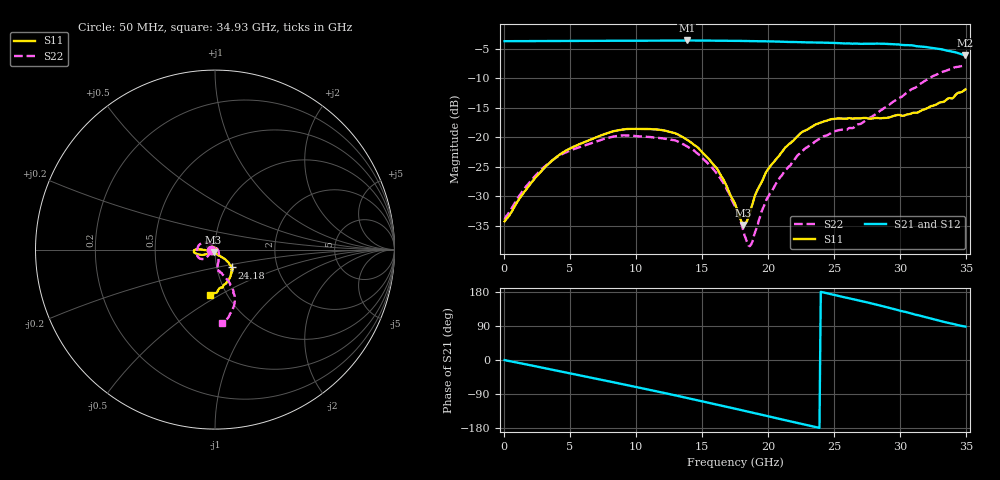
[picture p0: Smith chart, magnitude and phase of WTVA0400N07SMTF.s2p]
! 50 ohm 2-Port S-parameters measured by Modelithics Inc support@modelithics.com  Tampa, FL USA 813-866-6335 (February 2024)
! Smiths Interconnect,  4dB P/N: WTVA0400N07SMTF, Temperature: 50 C
! Board: 10 mil Rogers 4350B, Mounting Pad Dimensions: Length: 15 mils, Width: 25 mils, Gap: 40 mils.
# Hz S RI R 50
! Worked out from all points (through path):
!   352 points, 50 MHz to 34.93 GHz, reference 50 ohm
!   highest |S21| = -3.56 dB at 13.83 GHz (marker M1); lowest = -6.1 dB at 34.93 GHz (marker M2)
!   group delay of S21, straight-line fit = 21.7 ps
!   lowest |S11| = -34.9 dB at 18.11 GHz (marker M3), VSWR 1.04, Z = 49.2 - j1.58 ohm
!   |S11| at or under -10 dB: start of sweep to end of sweep
!   |S22| runs from -38.4 to -7.7 dB; largest |S21 - S12| = 0.0068
!   S11 on the Smith chart (normalised r, x): 50 MHz: 0.96, -0.00; 24.18 GHz: 1.18, -0.24; 34.93 GHz: 0.83, -0.45
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5e7  -0.0195 -0.000462  0.6541 -0.00359  0.6535 -0.00359  -0.0199 -0.00199
1.4935e9  -0.0301 -0.0157  0.6452 -0.1169  0.6447 -0.1168  -0.0289 -0.0217
2.8865e9  -0.0465 -0.0242  0.6176 -0.2259  0.6171 -0.2256  -0.0401 -0.0364
4.2795e9  -0.0662 -0.0293  0.5703 -0.3292  0.5696 -0.3291  -0.0531 -0.0472
5.8715e9  -0.0845 -0.0284  0.4946 -0.4358  0.4942 -0.4355  -0.0652 -0.0524
8.6575e9  -0.1135 -0.0182  0.3151 -0.5795  0.3141 -0.5792  -0.0944 -0.0416
1.1742e10  -0.1163 -0.00421  0.0674 -0.6576  0.0663 -0.657  -0.0989 0.00114
1.38315e10  -0.096 0.000931  -0.1156 -0.6535  -0.1159 -0.6528  -0.0772 0.0333
1.612e10  -0.0546 -0.00315  -0.3084 -0.5847  -0.3087 -0.5838  -0.0333 0.0361
1.7513e10  -0.0242 -0.0121  -0.4125 -0.5149  -0.4121 -0.5142  -0.00988 0.0238
1.811e10  -0.00825 -0.0161  -0.4526 -0.4762  -0.4518 -0.476  0.00129 0.0162
1.8508e10  0.00256 -0.021  -0.4768 -0.4506  -0.4767 -0.4498  0.0077 0.00936
1.8707e10  0.00734 -0.024  -0.4882 -0.4369  -0.488 -0.4361  0.011 0.00567
1.96025e10  0.0272 -0.0347  -0.5372 -0.3726  -0.5369 -0.3718  0.0209 -0.0139
2.05975e10  0.0456 -0.0467  -0.5806 -0.2916  -0.5801 -0.2911  0.0217 -0.0344
2.21895e10  0.0736 -0.0698  -0.6232 -0.1583  -0.6229 -0.1568  0.0201 -0.0668
2.33835e10  0.0876 -0.0892  -0.6365 -0.0542  -0.6358 -0.0543  0.0147 -0.0879
2.41795e10  0.0928 -0.0994  -0.6352 0.0188  -0.6346 0.0178  0.0137 -0.101
2.6468e10  0.0957 -0.1082  -0.5867 0.211  -0.5858 0.2111  0.0228 -0.1187
2.91545e10  0.095 -0.1132  -0.4577 0.4173  -0.4538 0.4204  0.0743 -0.1732
3.204e10  0.0826 -0.1562  -0.2172 0.5399  -0.2154 0.5399  0.11 -0.29
3.49255e10  -0.0276 -0.254  0.0149 0.4946  0.0144 0.4939  0.0388 -0.4092
